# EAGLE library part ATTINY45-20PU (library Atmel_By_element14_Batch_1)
8-bit Microcontroller with 2/4/8KBytes In-System Programmable Flash
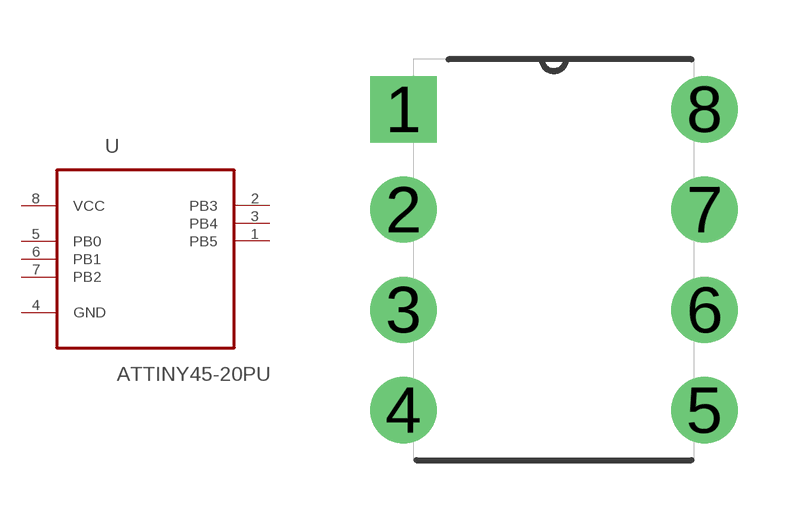
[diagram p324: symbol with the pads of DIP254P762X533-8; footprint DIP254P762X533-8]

Designator prefix U

## ATTINY45-20PU (MPN: ATTINY45-20PU; OC_FARNELL: 1288352; OC_NEWARK: 23M5072; PACKAGE: PDIP-8; SUPPLIER: Atmel)  [DIP254P762X533-8]
1  PB5
2  PB3
3  PB4
4  GND  pas
5  PB0
6  PB1
7  PB2
8  VCC  pwr

## Footprint DIP254P762X533-8 (pad centres in mm)
drill 1.118 square: 1 -7.62,7.62
drill 1.118: 2 -7.62,5.08; 3 -7.62,2.54; 4 -7.62,0; 5 0,0; 6 0,2.54; 7 0,5.08; 8 0,7.62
